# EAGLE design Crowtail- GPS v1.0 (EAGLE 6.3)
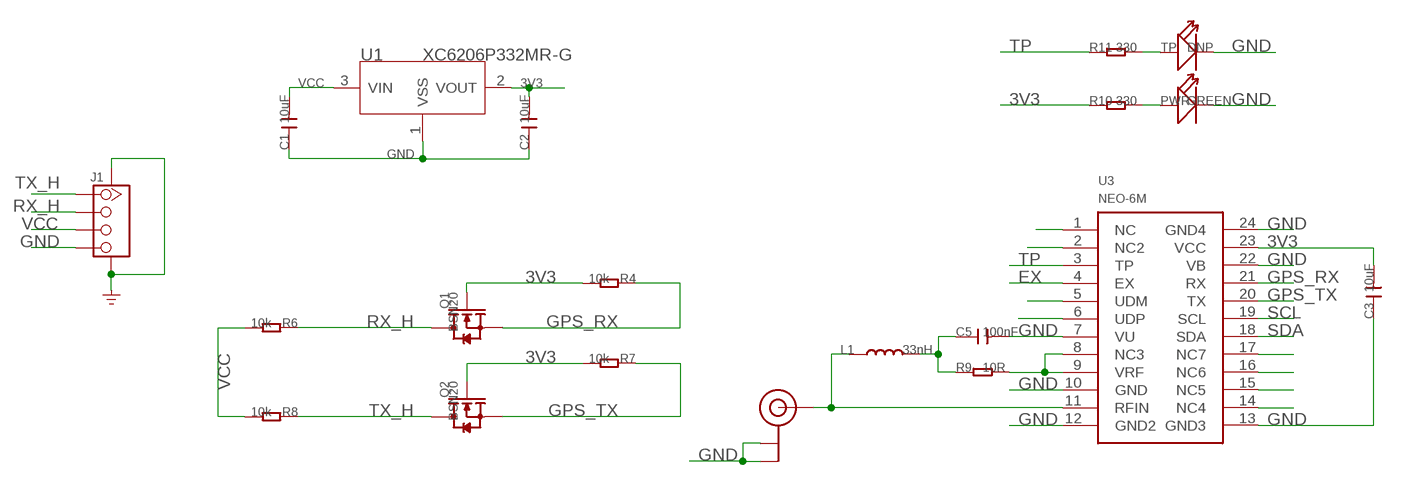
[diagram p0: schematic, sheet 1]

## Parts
C1  10uF  C-0603  [C0603]
C2  10uF  C-0603  [C0603]
C3  10uF  C-0603  [C0603]
C5  100nF  C-0603  [C0603]
J1  TWIG-4P-2.0-SMD-FEMALE-REINFORCE'90D'  [4P-SMD-2.0-90D]
L1  33nH  L'0603'  [L0603]
PWR  GREEN  LED'0603'  [LED-0603]
Q1  BSN20  MOSFET-N'SOT23'  [SOT23]
Q2  BSN20  MOSFET-N'SOT23'  [SOT23]
R4  10k  R-0603  [R0603]
R6  10k  R-0603  [R0603]
R7  10k  R-0603  [R0603]
R8  10k  R-0603  [R0603]
R9  10R  R-0603  [R0603]
R10  330  R-0603  [R0603]
R11  330  R-0603  [R0603]
TP  DNP  LED'0603'  [LED-0603]
U1  XC6206P332MR-G  XC6206MR  [SOT23]
U3  NEO-6M  [28P-1.1-16.0X12.2]
U4  U.FL  [U.FL]

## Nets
3V3: C2.2 C3.2 Q1.1(G) Q2.1(G) R4.2 R7.2 R10.1 U1.2(VOUT) U3.23(VCC)
EX: U3.4(EX)
GND: C1.1 C2.1 C3.1 C5.2 J1.4 J1.SS1 J1.SS2 PWR.- TP.- U1.1(VSS) U3.7(VU) U3.10(GND) U3.12(GND2) U3.13(GND3) U3.22(VB) U3.24(GND4) U4.P$1(GND) U4.P$2(GND)
GPS_RX: Q1.2(S) R4.1 U3.21(RX)
GPS_TX: Q2.2(S) R7.1 U3.20(TX)
N$1: U3.1(NC)
N$2: L1.1 U3.11(RFIN) U4.P$3(SIGNAL)
N$3: C5.1 L1.2 R9.1
N$4: U3.2(NC2)
N$5: U3.14(NC4)
N$6: PWR.+ R10.2
N$7: R9.2 U3.8(NC3) U3.9(VRF)
N$8: U3.15(NC5)
N$9: R11.2 TP.+
N$10: U3.16(NC6)
N$11: U3.17(NC7)
N$12: U3.5(UDM)
N$13: U3.6(UDP)
RX_H: J1.2 Q1.3(D) R6.1
SCL: U3.19(SCL)
SDA: U3.18(SDA)
TP: R11.1 U3.3(TP)
TX_H: J1.1 Q2.3(D) R8.1
VCC: C1.2 J1.3 R6.2 R8.2 U1.3(VIN)

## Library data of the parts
C1-C3 C5 = Discrete:C*: Ceramic Capacitors
J1 = Connector:TWIG-4P-2.0-SMD-FEMALE-REINFORCE
L1 = Discrete:L*
PWR TP = Discrete:LED*
Q1 Q2 = Discrete:MOSFET-N: IRLL014: http://www.vishay.com/docs/91319/sihll014.pdf
R4 R6-R11 = Discrete:R*
U1 = IC:XC6206: LOW ESR Cap.Compatible Positive Voltage Regulators
U3 = template:NEO-6M
U4 = SparkFun2:U.FL

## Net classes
0 default: width 0.003 mm, drill 0.254 mm, clearance 0.152 mm
3 usbvcc: width 0.203 mm, drill 0.305 mm, clearance 0.203 mm

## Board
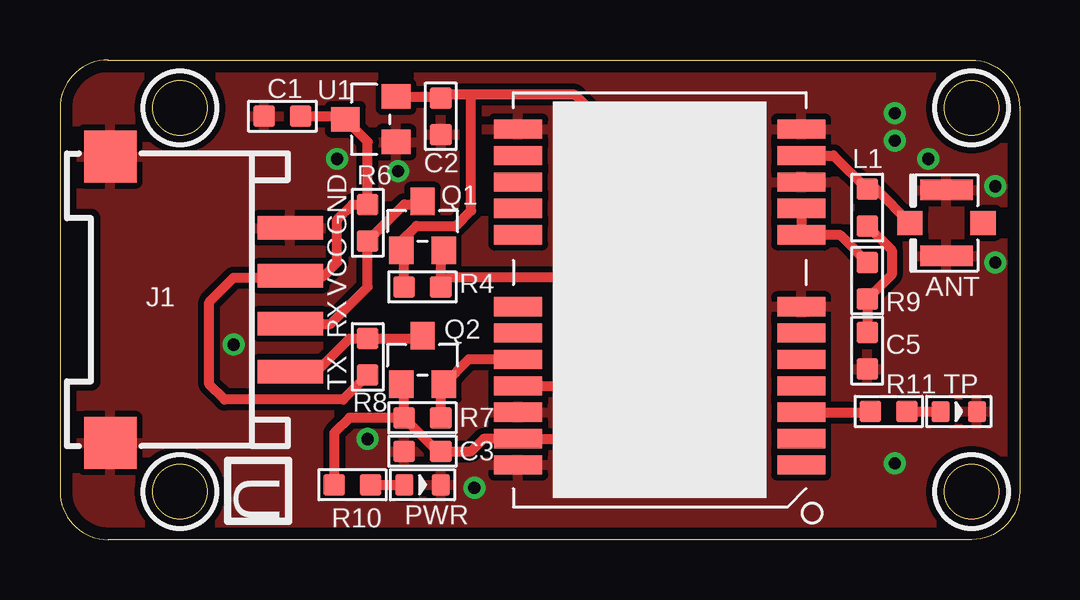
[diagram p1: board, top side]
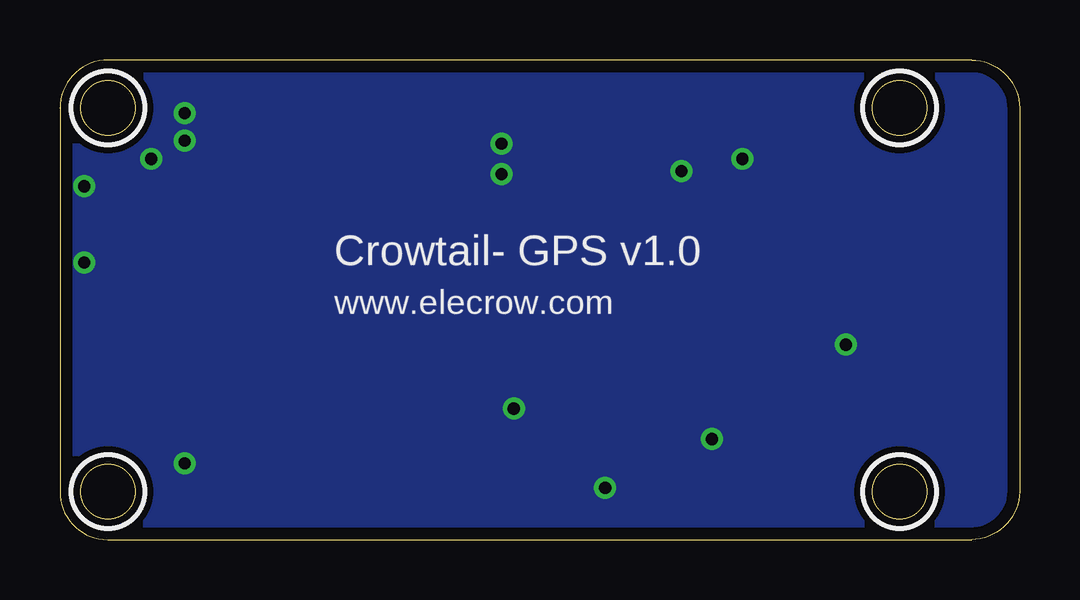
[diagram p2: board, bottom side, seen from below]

Size 40 x 20 mm. Coordinates in mm from the lower left corner, seen from the top.
Outline: 40,18 arc90 38,20 2,20 arc90 0,18 0,2 arc90 2,0 38.02,0 arc90 40,1.98 40,18
Outline: 40,18 40,18.02
Outline: circle at 5,18 radius 1.14
Outline: circle at 5,2 radius 1.14
Outline: circle at 38,18 radius 1.14
Outline: circle at 38,2 radius 1.14
Copper layers (1*16): Top 0.035mm / dielectric 1.5mm / Bottom 0.035mm
Design rules "default *": minimum track width 10mil, minimum drill 20mil, track to track 8mil, track to pad 8mil, pad to pad 8mil, via to via 8mil, smd to smd 8mil, copper to edge 20mil, drill to drill 8mil, minimum pad ring 10mil, minimum via ring 8mil, stop-mask expansion 2mil, vias tented up to drill 100mil, thermal gap 10mil
tRestrict: area 3.5,16.5 to 6.5,19.5; area 3.5,0.5 to 6.5,3.5; area 36.5,16.5 to 39.5,19.5; area 36.5,0.5 to 39.5,3.5
bRestrict: area 3.5,16.5 to 6.5,19.5; area 3.5,0.5 to 6.5,3.5; area 36.5,16.5 to 39.5,19.5; area 36.5,0.5 to 39.5,3.5

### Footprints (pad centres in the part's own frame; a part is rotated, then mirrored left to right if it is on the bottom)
C0603 = smd 0.889 x 0.889: 1 -0.762,0; 2 0.762,0
4P-SMD-2.0-90D = smd 0.965 x 2.74: 1 -3,-0.1; 2 -1,-0.1; 3 1,-0.1; 4 3,-0.1 | smd 2.159 x 2.184: SS1 -5.974,7.4; SS2 5.974,7.4
L0603 = smd 0.889 x 0.889: 1 -0.762,0; 2 0.762,0
LED-0603 = smd 0.762 x 0.889: + -0.762,0; - 0.762,0
SOT23 = smd 1.016 x 1.143: 1 -0.889,-1.016; 2 0.889,-1.016; 3 0,1.016
R0603 = smd 0.889 x 0.889: 1 -0.762,0; 2 0.762,0
SOT23' = smd 1.016 x 1.2: 1 -0.95,-1.06; 2 0.95,-1.06; 3 0,1.06
28P-1.1-16.0X12.2 = smd 2 x 0.8: 1 -5.904,6.888; 2 -5.904,5.788; 3 -5.904,4.688; 4 -5.904,3.588; 5 -5.904,2.488; 6 -5.904,1.388; 7 -5.904,0.288; 8 -5.904,-2.712; 9 -5.904,-3.812; 10 -5.904,-4.912; 11 -5.904,-6.012; 12 -5.904,-7.112; 13 5.896,-7.112; 14 5.896,-6.012; 15 5.896,-4.912; 16 5.896,-3.812; 17 5.896,-2.712; 18 5.896,0.288; 19 5.896,1.388; 20 5.896,2.488; 21 5.896,3.588; 22 5.896,4.688; 23 5.896,5.788; 24 5.896,6.888
U.FL = smd 2.2 x 0.85: P$1 0,1.375; P$2 0,-1.375 | smd 1.05 x 1: P$3 1.525,0; P$4 -1.525,0

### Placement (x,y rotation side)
C1  9.27,17.65 0 top
C2  15.88,17.65 90 top
C3  15.11,3.68 0 top
C5  33.66,7.87 270 top
J1  9.5,10 90 top
L1  33.66,13.84 270 top
PWR  15.11,2.29 0 top
Q1  15.11,13.08 0 top
Q2  15.11,7.49 0 top
R4  15.11,10.54 180 top
R6  12.83,13.21 90 top
R7  15.11,5.08 180 top
R8  12.83,7.62 270 top
R9  33.66,10.79 90 top
R10  12.19,2.29 0 top
R11  34.54,5.33 0 top
TP  37.47,5.33 0 top
U1  XC6206P332MR-G  [SOT23']  12.95,17.53 90 top
U3  25,10 180 top
U4  36.96,13.21 180 top

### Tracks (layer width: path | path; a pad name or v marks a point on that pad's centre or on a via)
3V3
  Top 0.406: R7.2 14.35,6.35 Q2.1 | R7.2 15.75,3.68 C3.2 17.14,3.68 17.65,4.19 19.08,4.19 | R7.2 12.06,5.08 11.43,4.45 R10.1 | R4.2 14.35,11.94 Q1.1 14.22,12.45 14.86,13.08 16.51,13.08 17.14,13.72 17.14,18.54 | U1.2 15.81,18.48 C2.2 16,18.54 17.14,18.54 | 19.08,4.19 U3.23 | 19.08,4.19 21.21,4.19 22.86,5.84 22.86,17.14 21.46,18.54 17.14,18.54
GND  (via drill 0.51)
  other vias: 34.8,17.78 21.59,16.51 11.56,15.88 34.8,3.17 21.08,5.46 17.27,2.16 12.83,4.19 21.59,15.24 7.24,8.13 34.8,16.64 38.99,14.73 36.2,15.88 38.99,11.56 14.1,15.37
  pour Top (isolate 0.254): -1.27,20.32 41.91,20.32 41.91,0.05 arc-90 41.86,0 -1.27,0
  pour Bottom (isolate 0.254): -1.27,20.32 41.91,20.32 41.91,0 -1.27,0
GPS_RX
  Top 0.406: U3.21 21.4,6.41 21.72,6.73 21.72,10.41 21.21,10.92 16.26,10.92 R4.1 15.88,11.94 Q1.2
GPS_TX
  Top 0.406: R7.1 15.88,6.35 Q2.2 17.04,7.51 U3.20
N$2
  Top 0.406: U3.11 32.25,16.01 L1.1 34.03,14.61 U4.P$3
N$3
  Top 0.406: L1.2 34.67,12.06 34.67,11.05 R9.1 C5.1
N$6
  Top 0.406: R10.2 PWR.+
N$7
  Top 0.406: U3.9 U3.8 32.5,12.71 R9.2
N$9
  Top 0.406: R11.2 TP.+
RX_H
  Top 0.406: Q1.3 14.99,13.97 14.35,13.97 R6.1 12.83,10.54 11.29,9 J1.2
TP
  Top 0.406: U3.3 33.76,5.31 R11.1
TX_H
  Top 0.406: J1.1 9.5,7.11 10.79,7.11 12.06,8.38 R8.1 14.99,8.38 Q2.3
VCC
  Top 0.406: C1.2 11.77,17.65 U1.3 12.83,16.59 R6.2 12.19,13.97 11.56,13.34 11.56,11.56 11,11 J1.3 9.42,10.92 7.24,10.92 6.22,9.91 6.22,6.48 6.86,5.84 11.81,5.84 R8.2

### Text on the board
tPlace: GND | VCC | ANT | RX | TX | U
bPlace: Crowtail- GPS v1.0 | www.elecrow.com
